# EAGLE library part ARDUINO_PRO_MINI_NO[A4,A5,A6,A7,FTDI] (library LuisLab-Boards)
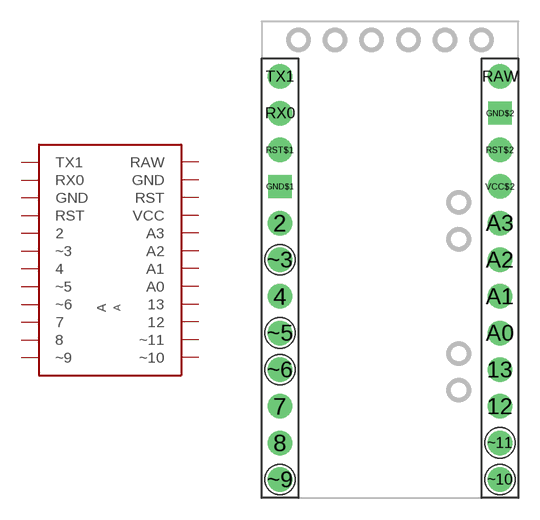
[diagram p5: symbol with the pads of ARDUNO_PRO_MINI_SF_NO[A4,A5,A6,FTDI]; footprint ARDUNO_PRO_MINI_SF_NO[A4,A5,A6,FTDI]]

Designator prefix A

## ARDUINO_PRO_MINI_NO[A4,A5,A6,A7,FTDI]  [ARDUNO_PRO_MINI_SF_NO[A4,A5,A6,FTDI]]
2  2
4  4
7  7
8  8
12  12
13  13
A0  A0
A1  A1
A2  A2
A3  A3
GND$1  GND
GND$2  GND
RAW  RAW
RST$1  RST
RST$2  RST
RX0  RX0
TX1  TX1
VCC$2  VCC
~3  ~3
~5  ~5
~6  ~6
~9  ~9
~10  ~10
~11  ~11

## Footprint ARDUNO_PRO_MINI_SF_NO[A4,A5,A6,FTDI] (pad centres in mm)
Arduino Pro Mini by SparkFun withoutA4, A5, A6, A7 and FTDI Serial TTL pads. Available in 5V and 3.3V versions.
drill 1.016 pad 1.7: 2 -7.62,2.54; 4 -7.62,-2.54; 7 -7.62,-10.16; 8 -7.62,-12.7; 12 7.62,-10.16; 13 7.62,-7.62; A0 7.62,-5.08; A1 7.62,-2.54; A2 7.62,0; A3 7.62,2.54; RAW 7.62,12.7; RST$1 -7.62,7.62; RST$2 7.62,7.62; RX0 -7.62,10.16; TX1 -7.62,12.7; VCC$2 7.62,5.08; ~3 -7.62,0; ~5 -7.62,-5.08; ~6 -7.62,-7.62; ~9 -7.62,-15.24; ~10 7.62,-15.24; ~11 7.62,-12.7
drill 1.016 pad 1.6 square: GND$1 -7.62,5.08; GND$2 7.62,10.16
